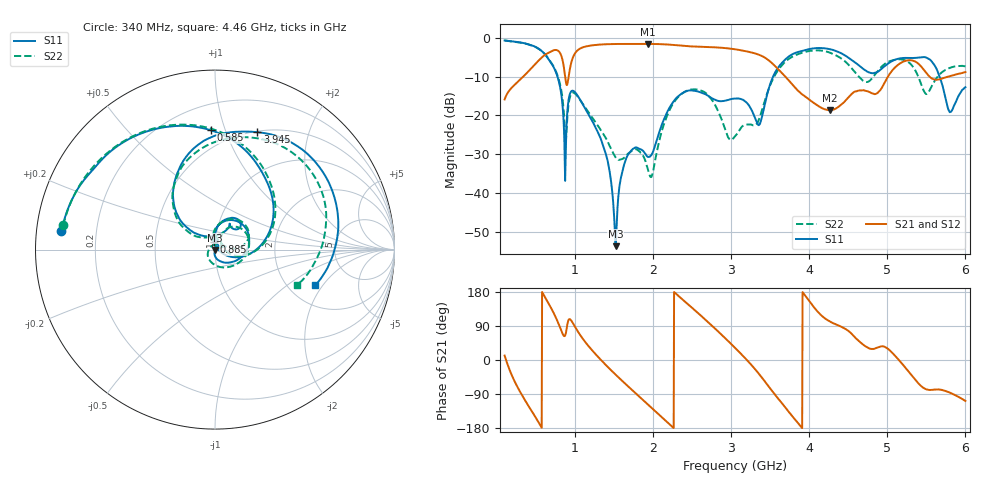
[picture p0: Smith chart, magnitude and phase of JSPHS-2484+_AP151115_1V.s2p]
!Mini-Circuits Laboratory
!S-Parameters
!Run/Lot/Date Code:MF33450/NA/1551
!Fixture/SN/Due: 90-4-20-21/70546/03/17/16
!Connection:PORT<IN> - pin<1>; PORT<OUT> - pin<7>;PORT<BIAS> - pin<4>;
!Tested With:PORT EXTENTION
!Network Analyzer:AG E5071C/74883/05/12/16
!Created: 01-07-2016 at 14:08:53
!MODEL: JSPHS-2484+
!S/N: V=1V
# MHZ S DB R 50
!Frequency  S11 dB  S11 DEG  S21 dB  S21 DEG  S12 dB  S12 DEG  S22 dB  S22 DEG
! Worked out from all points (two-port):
!   1181 points, 100 MHz to 6 GHz, reference 50 ohm
!   highest |S21| = -1.54 dB at 1.93 GHz (marker M1); lowest = -18.6 dB at 4.265 GHz (marker M2)
!   |S21| within 3 dB of the highest: 605.5 MHz to 825 MHz (219.5 MHz wide, 30.7 % of centre); 985.5 MHz to 3.381 GHz (2.395 GHz wide, 110 % of centre)
!   lowest |S11| = -53.7 dB at 1.52 GHz (marker M3), VSWR 1.00, Z = 50.2 - j0.137 ohm
!   |S11| at or under -10 dB: 777.3 MHz to 3.537 GHz (2.759 GHz wide, 128 % of centre); 5.669 GHz to end of sweep
!   |S22| runs from -35.9 to -0.7 dB; largest |S21 - S12| = 0.0044
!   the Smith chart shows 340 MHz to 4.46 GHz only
!   S11 on the Smith chart (normalised r, x): 340 MHz: 0.07, +0.06; 585 MHz: 0.38, +0.89; 885 MHz: 0.99, +0.09; 3.945 GHz: 0.51, +1.29; 4.46 GHz: 2.78, -1.70
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100  -0.64 -77.9  -15.87 11.7  -15.87 11.6  -0.66 -78.0
340  -1.29 173.1  -9.96 -98.9  -9.96 -99.0  -1.35 170.9
585  -3.55 91.9  -4.88 177.7  -4.88 177.7  -3.56 89.3
770  -9.55 21.1  -3.15 105.6  -3.15 105.6  -9.26 21.2
885  -27.16 96.3  -11.41 71.6  -11.41 71.6  -26.66 37.4
1085  -16.56 -18.0  -2.55 60.6  -2.55 60.6  -16.55 -30.6
1400  -30.24 -93.7  -1.61 -14.0  -1.61 -14.0  -26.00 -144.0
1520  -53.74 -41.5  -1.55 -38.4  -1.55 -38.4  -30.81 155.9
1670  -30.47 35.1  -1.54 -67.5  -1.54 -67.5  -30.10 66.5
1930  -30.66 38.3  -1.54 -116.4  -1.54 -116.4  -33.63 22.3
2070  -24.97 87.7  -1.58 -142.8  -1.58 -142.8  -27.43 102.1
2635  -14.22 42.7  -2.26 113.1  -2.26 113.1  -13.72 23.3
3050  -15.62 60.7  -2.92 32.2  -2.92 32.2  -25.41 67.9
3455  -15.01 142.0  -5.38 -62.7  -5.39 -62.7  -14.70 146.3
3945  -3.16 70.2  -15.04 171.0  -14.98 170.8  -3.62 70.9
4035  -2.74 56.8  -16.43 145.9  -16.40 145.6  -3.27 56.4
4265  -2.90 18.2  -18.59 101.5  -18.79 102.1  -3.80 16.4
4460  -4.53 -19.5  -16.23 82.8  -16.22 81.4  -6.05 -23.0
5020  -6.46 138.0  -9.59 27.5  -9.60 27.4  -6.09 106.6
5495  -5.04 23.3  -8.91 -77.1  -8.93 -77.3  -14.43 57.6
5800  -19.17 2.8  -9.85 -86.1  -9.87 -86.1  -7.74 71.8
6000  -12.70 27.4  -8.81 -108.0  -8.82 -108.0  -7.33 55.4
